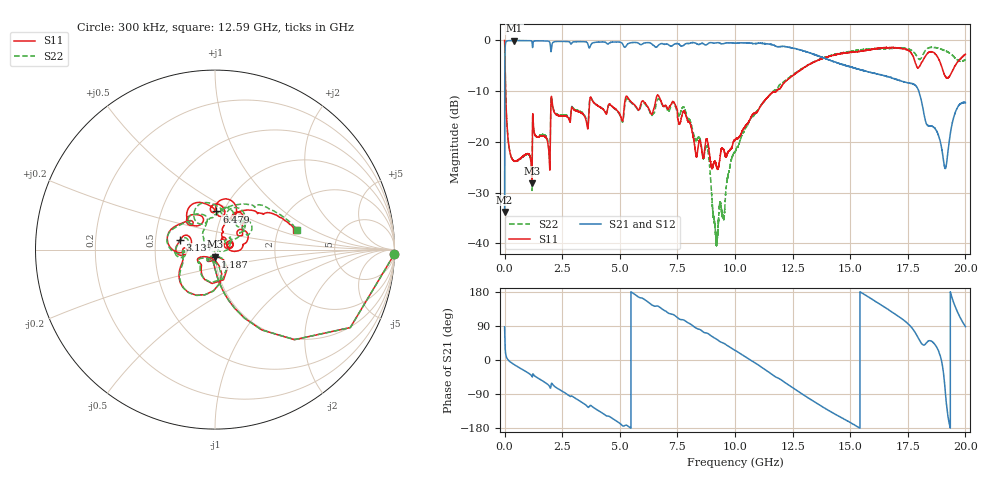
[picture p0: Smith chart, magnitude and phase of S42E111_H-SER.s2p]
! Created Wed Nov 25 21:56:06 2020
# khz S ma R 50
! 2 Port Network Data from SP1.SP block
! freq  magS11  angS11  magS21  angS21  magS12  angS12  magS22  angS22
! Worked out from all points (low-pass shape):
!   20001 points, 300 kHz to 20 GHz, reference 50 ohm
!   highest |S21| = -0.02 dB at 418.3 MHz (marker M1); lowest = -33.8 dB at 300 kHz (marker M2)
!   |S21| within 3 dB of the highest: 14.74 MHz to 13.61 GHz (13.59 GHz wide, 200 % of centre); 13.60983 GHz to 13.61048 GHz (650.1 kHz wide, 0.00478 % of centre)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
!   lowest |S11| = -28.2 dB at 1.186 GHz (marker M3), VSWR 1.08, Z = 49.9 - j3.9 ohm
!   |S11| at or under -10 dB: 44.34 MHz to 11.79 GHz (11.75 GHz wide, 199 % of centre)
!   |S22| runs from -40.5 to 0.0 dB; largest |S21 - S12| = 0.015
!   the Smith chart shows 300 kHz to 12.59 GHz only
!   S11 on the Smith chart (normalised r, x): 300 kHz: 1, -81; 1.187 GHz: 1.00, -0.08; 3.137 GHz: 0.67, +0.07; 6.479 GHz: 0.93, +0.41; 12.59 GHz: 2.51, +0.70
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300  0.9997 -1.4  0.02047 87.7  0.02057 88.6  0.9992 -1.5
106300  0.1434 -85.9  0.989 4.3  0.9888 4.2  0.1442 -86.1
418300  0.06489 -102.0  0.9978 -12.2  0.9972 -12.2  0.06499 -102.9
1186300  0.03907 -89.9  0.9745 -43.0  0.9747 -43.0  0.03356 -97.8
1187300  0.03911 -86.5  0.9726 -43.2  0.9725 -43.2  0.03355 -93.8
3137300  0.2016 164.7  0.9727 -103.6  0.972 -103.5  0.2056 169.4
3334300  0.1932 157.6  0.9732 -110.8  0.972 -110.8  0.1968 162.5
4965300  0.1937 110.9  0.9639 -165.6  0.9646 -165.7  0.1909 104.7
6479300  0.2129 87.8  0.8905 142.8  0.8901 142.8  0.192 67.3
6667300  0.2879 72.1  0.892 142.0  0.8906 142.0  0.2666 59.0
8783300  0.1063 17.1  0.9127 71.0  0.9129 71.1  0.08998 22.3
9179300  0.05936 31.9  0.946 55.7  0.9456 55.7  0.01036 -47.0
1.00003e7  0.1052 64.5  0.9401 25.4  0.9401 25.5  0.07975 142.0
1.11563e7  0.234 60.8  0.9358 -19.2  0.9341 -19.1  0.233 77.8
1.25893e7  0.4658 13.6  0.8333 -76.7  0.8368 -76.5  0.4728 13.2
1.33343e7  0.5962 -13.8  0.742 -106.2  0.7471 -106.1  0.6005 -18.6
1.50603e7  0.7643 -78.5  0.5451 -166.7  0.5449 -167.4  0.784 -75.1
1.66673e7  0.8488 -136.8  0.4392 132.6  0.4294 133.2  0.8352 -134.8
1.78913e7  0.5513 176.7  0.3475 65.2  0.3521 65.2  0.7004 176.3
1.85043e7  0.7748 171.3  0.1437 50.2  0.1443 50.6  0.8549 164.8
1.91163e7  0.4487 146.9  0.05524 -75.1  0.05481 -75.7  0.7946 141.4
2e7  0.7327 147.7  0.2439 88.1  0.2474 88.6  0.646 129.8
